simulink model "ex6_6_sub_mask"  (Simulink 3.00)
settings: Solver=ode15s  SolverMode=SingleTasking  StartTime=0.0  StopTime=1000  RelTol=1e-3  AbsTol=1e-6
libraries: simulink3 x1

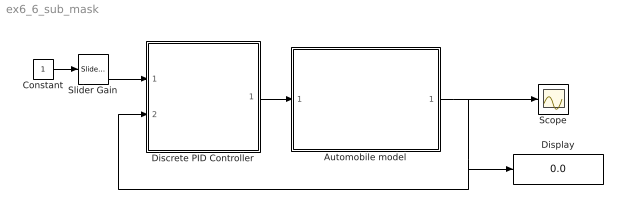
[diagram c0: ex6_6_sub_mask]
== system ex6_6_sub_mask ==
  Automobile model : Subsystem
  Constant : Constant  Value=1
  Discrete PID Controller : Subsystem  mask(Moj blok){kp=50, ki=0.75}
      mask prompts: kp "ojac. prop. dela:"; ki "Ojac. int. dela:"
      mask help: Opis
  Display : Display
  Scope : Scope
  Slider Gain : simulink3/Math/Slider Gain  low=0  gain=50  high=100
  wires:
  Discrete PID Controller/1(Commanded Thrust) -> Automobile model/1(Commanded Thrust)
  Constant/1 -> Slider Gain/1
  Slider Gain/1 -> Discrete PID Controller/1(Desired speed)
  Automobile model/1(Speed Out) -> Scope/1, Discrete PID Controller/2(Actual speed), Display/1

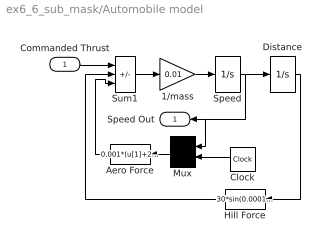
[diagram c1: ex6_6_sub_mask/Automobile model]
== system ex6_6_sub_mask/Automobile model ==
  Commanded Thrust : Inport  Port=1  PortWidth=-1  SampleTime=0  DataType=auto
  1/mass : Gain  Gain=0.01  SaturateOnIntegerOverflow=on
  Aero Force : Fcn  Orientation=left  Expr=0.001*(u[1]+20*sin(0.01*u[2]))^2
  Clock : Clock
  Distance : Integrator  ExternalReset=none  InitialConditionSource=internal  InitialCondition=0  LimitOutput=off  UpperSaturationLimit=inf  LowerSaturationLimit=-inf  ShowSaturationPort=off  ShowStatePort=off  AbsoluteTolerance=auto
  Hill Force : Fcn  Orientation=left  Expr=30*sin(0.0001*u[1])
  Mux : Mux  Orientation=left  Inputs=2
  Speed : Integrator  ExternalReset=none  InitialConditionSource=internal  InitialCondition=0  LimitOutput=off  UpperSaturationLimit=inf  LowerSaturationLimit=-inf  ShowSaturationPort=off  ShowStatePort=off  AbsoluteTolerance=auto
  Sum1 : Sum  Inputs=+--  SaturateOnIntegerOverflow=on
  Speed Out : Outport  Orientation=left  Port=1
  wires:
  Speed/1 -> Distance/1, Mux/1, Speed Out/1
  Clock/1 -> Mux/2
  1/mass/1 -> Speed/1
  Sum1/1 -> 1/mass/1
  Distance/1 -> Hill Force/1
  Hill Force/1 -> Sum1/2
  Aero Force/1 -> Sum1/3
  Mux/1 -> Aero Force/1
  Commanded Thrust/1 -> Sum1/1

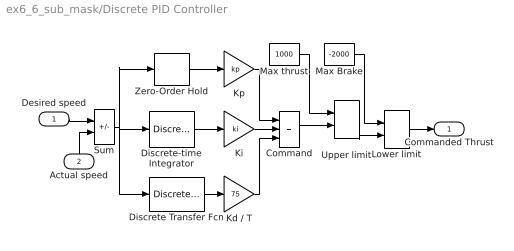
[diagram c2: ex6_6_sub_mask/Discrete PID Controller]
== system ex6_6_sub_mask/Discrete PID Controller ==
  Desired speed : Inport  Port=1  PortWidth=-1  SampleTime=0.5  DataType=auto
  Actual speed : Inport  Orientation=up  Port=2  PortWidth=-1  SampleTime=0.5  DataType=auto
  Command : Sum  Inputs=+++  SaturateOnIntegerOverflow=on
  Discrete Transfer Fcn : DiscreteTransferFcn  Numerator=[1 -1]  Denominator=[1 0]  SampleTime=0.5
  Discrete-time Integrator : DiscreteIntegrator  IntegratorMethod=ForwardEuler  ExternalReset=none  InitialConditionSource=internal  InitialCondition=0  LimitOutput=on  UpperSaturationLimit=100  LowerSaturationLimit=-100  ShowSaturationPort=off  ShowStatePort=off  SampleTime=0.5
  Kd / T : Gain  Gain=75  SaturateOnIntegerOverflow=on
  Ki : Gain  Gain=ki  SaturateOnIntegerOverflow=on
  Kp : Gain  Gain=kp  SaturateOnIntegerOverflow=on
  Lower limit : MinMax  Function=max  Inputs=2
  Max Brake : Constant  Value=-2000
  Max thrust : Constant  Value=1000
  Sum : Sum  Inputs=+-  SaturateOnIntegerOverflow=on
  Upper limit : MinMax  Function=min  Inputs=2
  Zero-Order Hold : ZeroOrderHold  SampleTime=0.5
  Commanded Thrust : Outport  Port=1
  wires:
  Actual speed/1 -> Sum/2
  Max Brake/1 -> Lower limit/1
  Max thrust/1 -> Upper limit/1
  Upper limit/1 -> Lower limit/2
  Zero-Order Hold/1 -> Kp/1
  Discrete-time Integrator/1 -> Ki/1
  Sum/1 -> Discrete-time Integrator/1, Zero-Order Hold/1, Discrete Transfer Fcn/1
  Discrete Transfer Fcn/1 -> Kd / T/1
  Kp/1 -> Command/1
  Ki/1 -> Command/2
  Kd / T/1 -> Command/3
  Command/1 -> Upper limit/2
  Desired speed/1 -> Sum/1
  Lower limit/1 -> Commanded Thrust/1
